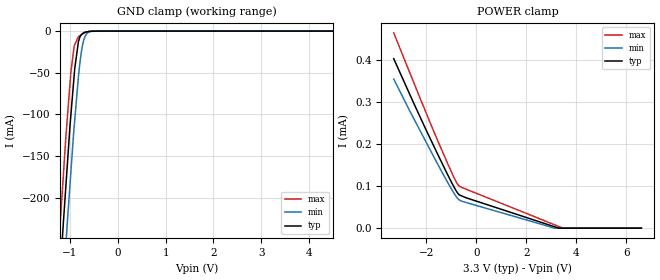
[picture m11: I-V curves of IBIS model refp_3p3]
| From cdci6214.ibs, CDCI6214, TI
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|   refp_3p3 Model
[Model]   refp_3p3
Model_type   Input
Vinl = 0.66
Vinh = 2.64
|   typ   min   max
C_comp   7.326E-13   6.929E-13   7.752E-13
|  Where Nom  PVT is Nominal Process, 3.3V,   32C
|   Fast PVT is Strong Process,  3.465V, -35C
|   Slow PVT is Weak Process,   3.135V,  110C
[Model spec]
|subparameter
Vinl   0.66   0.627   0.693
Vinh   2.64   2.508   2.772
[Voltage Range]   3.3   3.135   3.465
|Junction Temperature
[Temperature Range]   32   110   -35
[Power Clamp Reference]   3.3   3.135   3.465
[GND Clamp Reference]   0   0   0
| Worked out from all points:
|   GND clamp passes 1 mA (typ) near -0.65 V on its own axis
[GND Clamp]
|   Voltage   I(typ)   I(min)   I(max)
-3.3V     -2.319A    -2.382A    -2.268A
-1.236V   -318.5mA   -389.4mA   -258.8mA
-1.146V   -236.1mA   -309.3mA   -179.3mA
-1.087V   -186.9mA   -257.5mA   -127.8mA
-1.055V   -159.9mA   -229mA     -103.9mA
-982.4mV  -101.3mA   -169.9mA   -49.78mA
-901.4mV  -45.1mA    -107.1mA   -16.34mA
-794.8mV  -7.458mA   -39.14mA   -5.586mA
-741.3mV  -3.112mA   -17.94mA   -3.782mA
-683.6mV  -1.28mA    -6.216mA   -1.832mA
-348.3mV  -7.822uA   -9.936uA   -8.696uA
6.6V      0A         0A         0A
[POWER Clamp]
|   Voltage   I(typ)   I(min)   I(max)
-3.3V     402.9uA    354.4uA    464.2uA
-2.482V   294.9uA    258.8uA    343.8uA
-1.481V   168.3uA    145.6uA    199.8uA
-956.6mV  105.3uA    89.33uA    129uA
-763.6mV  85.16uA    72.15uA    106.1uA
-672.5mV  78.93uA    66.95uA    99.61uA
-400.4mV  72.09uA    60.93uA    92.57uA
3.134V    3.239uA    10.33nA    7.94uA
3.299V    607.7pA    0A         3.964uA
3.464V    0A         0A         15.92nA
6.6V      0A         0A         0A
